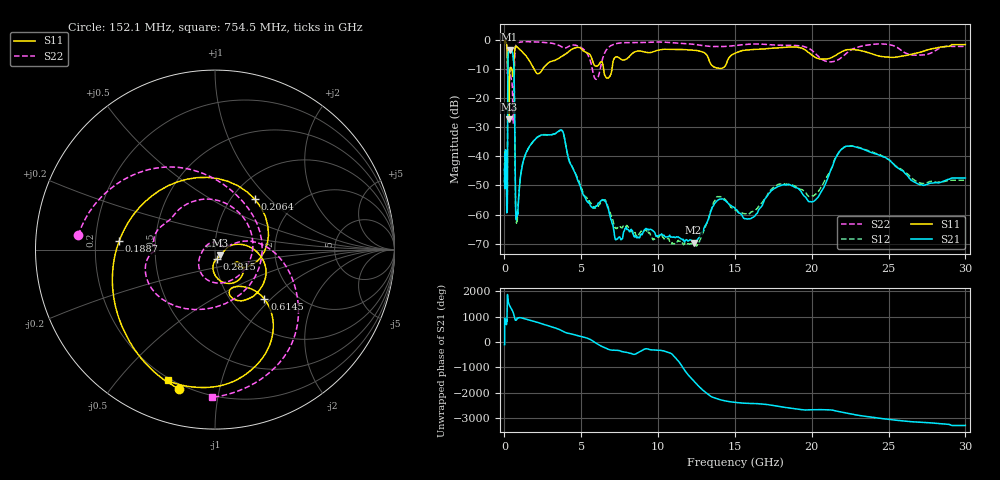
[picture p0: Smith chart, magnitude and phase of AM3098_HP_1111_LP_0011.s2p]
! Date/Time: Thu, Feb 28, 2019 8:47 AM
! Network Analyzer: Agilent Technologies E8364B Rev: A.07.50.67
! Sweep from 0.010 to 30.000 GHz, 1601 Points, Sweep Type: LOG
! Power Supply: 5.022 V, 0.002 A
# Hz S DB R 50
!freq MagS11 AngS11 MagS21 AngS21 MagS12 AngS12 MagS22 AngS22
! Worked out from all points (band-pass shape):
!   1601 points, 10 MHz to 30 GHz, reference 50 ohm
!   highest |S21| = -3.38 dB at 332.1 MHz (marker M1); lowest = -69.6 dB at 12.31 GHz (marker M2)
!   |S21| within 3 dB of the highest: 228.2 MHz to 581.6 MHz (353.5 MHz wide, 87.3 % of centre)
!   lowest |S11| = -27.3 dB at 288.7 MHz (marker M3), VSWR 1.09, Z = 53 - j3.28 ohm
!   |S11| at or under -10 dB: 210 MHz to 363.4 MHz (153.4 MHz wide, 53.5 % of centre); 1.92 GHz to 2.495 GHz (575 MHz wide, 26 % of centre); 6.45 GHz to 7.001 GHz (551.1 MHz wide, 8.19 % of centre)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
!   |S22| runs from -28.6 to -0.5 dB; largest |S21 - S12| = 0.013
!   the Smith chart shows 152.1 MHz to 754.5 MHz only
!   S11 on the Smith chart (normalised r, x): 152.1 MHz: 0.18, -0.76; 188.7 MHz: 0.30, +0.04; 206.4 MHz: 1.28, +0.82; 281.5 MHz: 1.01, -0.11; 614.5 MHz: 1.41, -0.92; 754.5 MHz: 0.19, -0.69
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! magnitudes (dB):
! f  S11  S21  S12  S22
! 10 MHz  -0.3  -44.8  -43.0  -0.5
! 38.04 MHz  -0.2  -41.2  -40.8  -0.6
! 96 MHz  -0.8  -39.3  -39.8  -1.2
! 144.7 MHz  -1.6  -57.0  -54.8  -2.0
! 152.1 MHz  -1.9  -59.2  -56.0  -2.3
! 188.7 MHz  -5.4  -55.5  -51.6  -9.2
! 206.4 MHz  -8.9  -21.8  -21.7  -9.1
! 281.5 MHz  -25.6  -3.7  -3.6  -9.8
! 288.7 MHz  -27.3  -3.6  -3.5  -10.1
! 332.1 MHz  -12.4  -3.4  -3.4  -10.4
! 550.5 MHz  -12.6  -5.1  -5.0  -26.1
! 614.5 MHz  -8.2  -9.7  -9.7  -18.5
! 754.5 MHz  -2.2  -60.4  -61.1  -1.7
! 2.084 GHz  -11.4  -33.6  -33.7  -0.7
! 3.723 GHz  -5.8  -31.0  -31.1  -2.4
! 5.959 GHz  -9.1  -57.0  -57.6  -13.6
! 7.926 GHz  -6.6  -64.4  -63.9  -1.0
! 12.31 GHz  -3.6  -69.6  -70.3  -1.5
! 13.95 GHz  -9.8  -54.9  -53.9  -2.3
! 20.1 GHz  -5.6  -55.5  -53.6  -4.0
! 22.56 GHz  -3.3  -36.4  -36.4  -3.5
! 30 GHz  -1.7  -47.4  -48.2  -2.3
